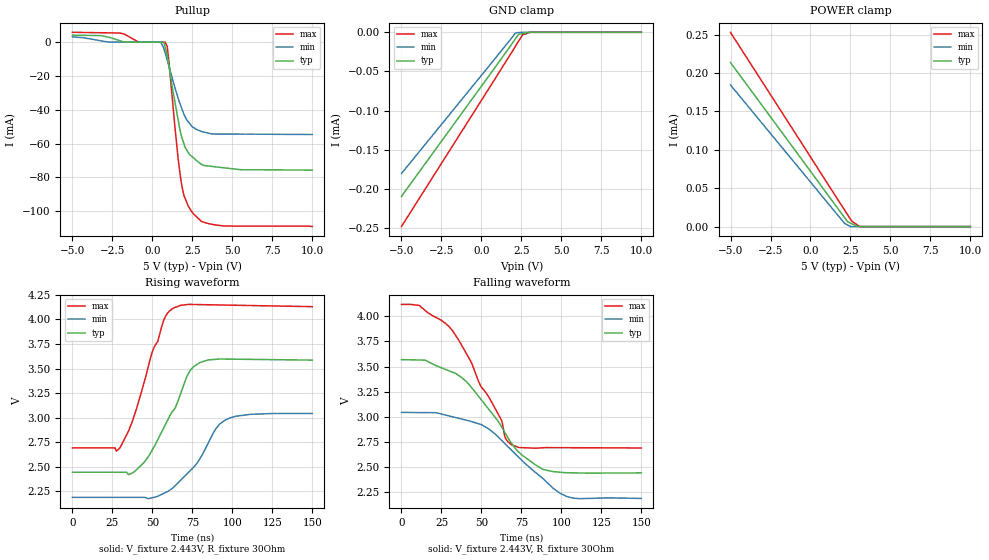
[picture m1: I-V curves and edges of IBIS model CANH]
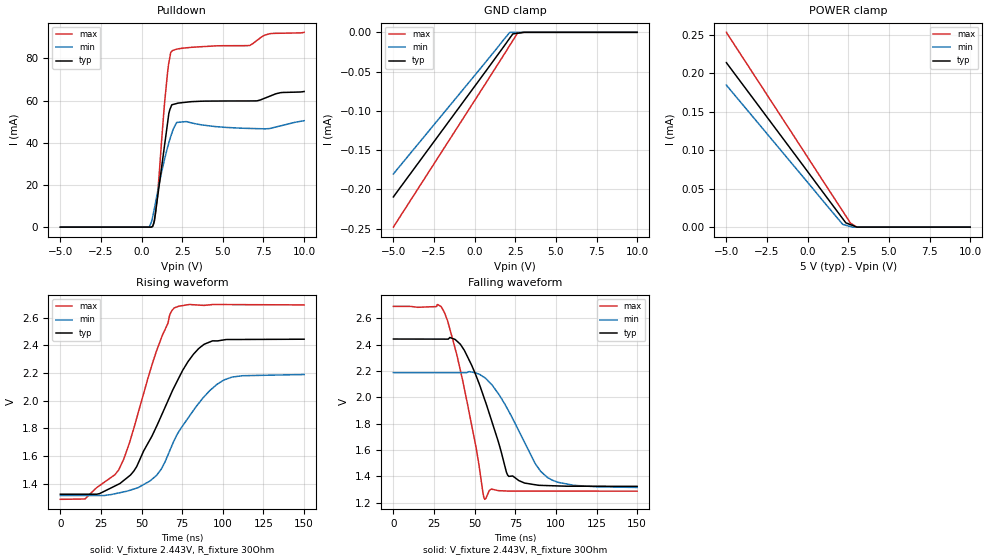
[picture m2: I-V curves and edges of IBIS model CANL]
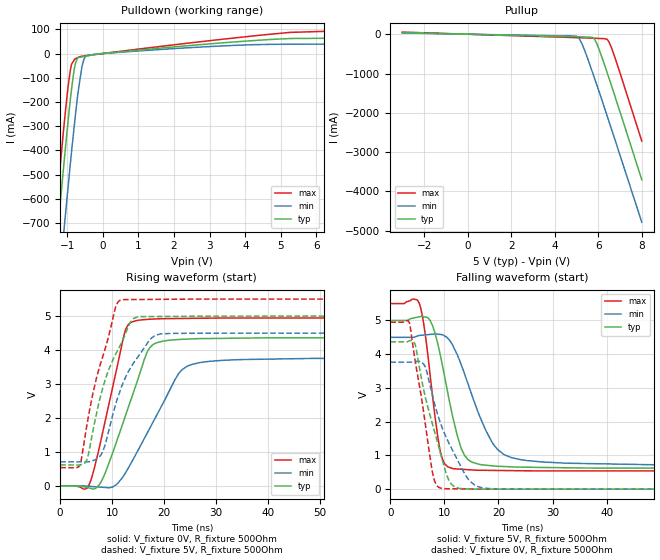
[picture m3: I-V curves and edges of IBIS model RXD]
|Texas Instruments Incorporated
|Automotive Fault Protected CAN Transceiver With Flexible Data-Rate
|Marketing part#   Digital Voltage Range   Package-type   #pins
|TCAN1044D   4.5-5.5V   SOIC   8
[IBIS Ver]   3.2
[File name]   tcan1044-q1.ibs
[File Rev]   1.0
[Date]   11/06/2019
[Source]
| Texas Instruments Incorporated.
| 12500 TI Blvd
| Dallas, TX -75243
[Notes]   Revision History:
| Rev 1.0: 11/06/2019
| - Initial version of the model
| - Model generated from simulations in SPECTRE
| - Model matched to SPICE simulation
| - C_comp although listed in numerical order of value are
|   obtained from varying PVT conditions. For PVT conditions for
|   each specific value refer the buffer description under
|   respective [Model]. IBIS model user is responsible for using
|   appropriate C_comp to simulate for Signal Integrity.
| - Warnings regarding combined Non-monotonicity of various models have been
| reviewed and considered minor and can be ignored.
|* EXCEPTION:   *
|* - For models RXD pullup and pulldown IV curves do not pass   *
|*   through zero because of resistors connected to pad.   *
|* - For CANH model pullup table does not pass through zero   *
|*   due to resistor network connected to PAD. Power clamp table has   *
|*   leakage due to resistor network connected to PAD   *
|* - For CANL model pulldown table does not pass through zero   *
|*   due to resistor network connected to PAD. Power clamp table has   *
|*   leakage due to resistor network connected to PAD   *
[Disclaimer]
| This model is designed as an aid for customers of Texas Instruments.
| TI and its licensors and suppliers make no warranties, either expressed
| or implied, with respect to this  model, including the warranties of
| merchantability or fitness for a particular purpose. The model is
| provided solely on an "as is" basis. The entire risk as to its quality
| and performance is with the customer.
[Copyright]
(C) Copyright 2019 Texas Instruments Incorporated.All rights reserved.
|   TCAN1044D
[Component]   TCAN1044D
[Manufacturer]   TI
[Package]   |8 SOIC - D Package
|   typ   min   max
R_pkg   0.068   0.038   0.098
L_pkg   2.235nH   1.713nH   2.756nH
C_pkg   0.393pF   0.337pF   0.449pF
[Pin]  signal_name   model_name   R_pin   L_pin   C_pin
1   TXD   TXD   0.093   2.653n   0.337p
2   GND   GND   0.038   1.716n   0.449p
3   VCC   POWER   0.038   1.713n   0.449p
4   RXD   RXD   0.093   2.657n   0.337p
5   VIO   POWER   0.098   2.756n   0.341p
6   CANL   CANL   0.092   2.624n   0.363p
7   CANH   CANH   0.075   2.301n   0.349p
8   STB   STB   0.094   2.677n   0.338p
[Diff_pin]   inv_pin   vdiff   tdelay_typ   tdelay_min   tdelay_max
7   6   NA   NA   NA   NA
| Models and submodels in the file (5): CANH (I/O_open_source), CANL (I/O_open_drain), RXD (Output), STB (Input), TXD (Input)
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|   CANH Model
[Model]   CANH
Model_type   I/O_open_source
Polarity   Inverting
Enable   Active-Low
Vinl = 0.5
Vinh = 0.9
Vmeas = 3
Vref = 2.443
Cref = 2pF
Rref = 30
|   typ   min   max
C_comp   12.2e-12   11.49e-12   12.57e-12
[Voltage Range]   5   4.5   5.5
[Temperature Range]   25   150   -55
[Pullup Reference]   5   4.5   5.5
[Pulldown Reference]   0   0   0
[Power Clamp Reference]   5   4.5   5.5
[GND Clamp Reference]   0   0   0
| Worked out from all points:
|   slope of the pullup table from 0 to 0.75 V, typ, clamps not added: 727 ohm
|   falling waveform, V_fixture 2.443V, R_fixture 30Ohm: 20-80 % time 31.2ns typ, 35.1ns min, 29.3ns max; typ from 3.57 V to 2.44 V
|   rising waveform, V_fixture 2.443V, R_fixture 30Ohm: 20-80 % time 20.2ns typ, 21.6ns min, 16.6ns max; typ from 2.44 V to 3.59 V
[GND Clamp]
|   Voltage   I(typ)   I(min)   I(max)
-5V       -209.7uA   -180.5uA   -248.2uA
2.128V    -8.187uA   -910.9nA   -17.7uA
2.322V    -2.722uA   -432nA     -11.25uA
2.569V    -1.686uA   0A         -3.295uA
3.064V    0A         0A         0A
10V       0A         0A         0A
[Pullup]
|   Voltage   I(typ)   I(min)   I(max)
-5V       4.168mA    3.187mA    5.861mA
-2.061V   962.1uA    55.5uA     5.435mA
-861.1mV  8.134uA    7.958uA    128.5uA
482.5mV   3.073uA    -99.63uA   3.64uA
797.2mV   -2.85mA    -6.239mA   -7.214uA
930.8mV   -8.028mA   -10.68mA   -2.658mA
1.594V    -45.06mA   -32.61mA   -67.39mA
1.848V    -56.59mA   -39.51mA   -85.28mA
2.229V    -65.02mA   -46.88mA   -96.72mA
3.064V    -72.18mA   -52.81mA   -106mA
4.442V    -74.24mA   -54.38mA   -108.7mA
10V       -75.66mA   -54.59mA   -109mA
[POWER Clamp]
|   Voltage   I(typ)   I(min)   I(max)
-5V       213.6uA    184.5uA    252.9uA
2.128V    11.78uA    4.269uA    21.63uA
2.322V    6.298uA    2.025uA    15.35uA
2.569V    3.9uA      0A         7.37uA
3.064V    0A         0A         0A
10V       0A         0A         0A
[Ramp]
R_load = 30
|   typ   min   max
dV/dt_r   0.685442/2.00542e-08   0.512592/2.14191e-08   0.863536/1.66139e-08
dV/dt_f   0.674704/3.11586e-08   0.512317/3.5057e-08   0.855212/2.92131e-08
[Falling Waveform]
V_fixture = 2.443V
V_fixture_min = 2.188V
V_fixture_max = 2.691V
R_fixture = 30Ohm
C_fixture = 0F
|   Time   V(typ)   V(min)   V(max)
0s        3.569V     3.045V     4.117V
11.28ns   3.565V     3.043V     4.106V
31.67ns   3.445V     3.002V     3.861V
50.06ns   3.167V     2.923V     3.294V
62.3ns    2.909V     2.772V     2.975V
64.87ns   2.84V      2.731V     2.793V
68.51ns   2.745V     2.674V     2.726V
88.48ns   2.479V     2.388V     2.694V
103.4ns   2.446V     2.21V      2.694V
150ns     2.444V     2.191V     2.691V
[Rising Waveform]
V_fixture = 2.443V
V_fixture_min = 2.188V
V_fixture_max = 2.691V
R_fixture = 30Ohm
C_fixture = 0F
|   Time   V(typ)   V(min)   V(max)
0s        2.443V     2.188V     2.691V
29.42ns   2.443V     2.188V     2.686V
37.65ns   2.437V     2.188V     2.97V
45.02ns   2.548V     2.188V     3.371V
57.13ns   2.897V     2.228V     3.994V
62.96ns   3.071V     2.285V     4.115V
75.77ns   3.519V     2.493V     4.153V
89.67ns   3.594V     2.888V     4.148V
95.81ns   3.596V     2.978V     4.147V
150ns     3.586V     3.042V     4.13V
|   CANL Model
[Model]   CANL
Model_type   I/O_open_drain
Polarity   Non-Inverting
Enable   Active-Low
Vinl = 0.5
Vinh = 0.9
Vmeas = 2
Vref = 2.443
Cref = 2pF
Rref = 30
|   typ   min   max
C_comp   11.96e-12   11.44e-12   12.21e-12
[Voltage Range]   5   4.5   5.5
[Temperature Range]   25   150   -55
[Pullup Reference]   5   4.5   5.5
[Pulldown Reference]   0   0   0
[Power Clamp Reference]   5   4.5   5.5
[GND Clamp Reference]   0   0   0
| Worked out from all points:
|   slope of the pulldown table from 0 to 0.75 V, typ, clamps not added: 373 ohm
|   falling waveform, V_fixture 2.443V, R_fixture 30Ohm: 20-80 % time 18.1ns typ, 22.3ns min, 14.4ns max; typ from 2.44 V to 1.32 V
|   rising waveform, V_fixture 2.443V, R_fixture 30Ohm: 20-80 % time 27.4ns typ, 26.3ns min, 22.2ns max; typ from 1.32 V to 2.44 V
[Pulldown]
|   Voltage   I(typ)   I(min)   I(max)
-5V       30fA       -53.22pA   460fA
252.8mV   4.719uA    -3.121uA   -1.871uA
647.3mV   194.8uA    3.573mA    145.6uA
782.7mV   2.825mA    8.677mA    2.945mA
979mV     13.95mA    16.53mA    15.09mA
1.407V    38.49mA    32.05mA    58.45mA
1.6V      49.55mA    37.9mA     73.56mA
1.894V    58.11mA    45.29mA    83.7mA
2.755V    59.27mA    50.08mA    85.07mA
6.669V    59.86mA    46.81mA    86.22mA
7.601V    61.23mA    46.63mA    91.14mA
10V       64.34mA    50.49mA    92.41mA
[GND Clamp]
|   Voltage   I(typ)   I(min)   I(max)
-5V       -209.7uA   -180.5uA   -248.2uA
2.155V    -7.531uA   -153.4nA   -16.77uA
2.349V    -2.037uA   -103.9nA   -10.51uA
2.638V    -1.181uA   -29.97nA   -1.117uA
3.037V    0A         0A         0A
10V       0A         0A         0A
[POWER Clamp]
|   Voltage   I(typ)   I(min)   I(max)
-5V       213.6uA    184.5uA    252.9uA
2.155V    11.02uA    3.595uA    20.77uA
2.349V    5.558uA    2.436uA    14.52uA
2.638V    3.222uA    702.3nA    5.157uA
3.031V    53.18nA    0A         0A
10V       0A         0A         0A
[Ramp]
R_load = 30
|   typ   min   max
dV/dt_r   0.671493/2.72876e-08   0.524178/2.61335e-08   0.842197/2.20483e-08
dV/dt_f   0.671494/1.80697e-08   0.523421/2.22127e-08   0.842202/1.44627e-08
[Falling Waveform]
V_fixture = 2.443V
V_fixture_min = 2.188V
V_fixture_max = 2.691V
R_fixture = 30Ohm
C_fixture = 0F
|   Time   V(typ)   V(min)   V(max)
0s        2.443V     2.188V     2.691V
27.22ns   2.443V     2.188V     2.706V
31.4ns    2.443V     2.188V     2.646V
41.22ns   2.404V     2.188V     2.205V
56.2ns    1.983V     2.15V      1.226V
60.2ns    1.832V     2.101V     1.303V
71.01ns   1.4V       1.894V     1.288V
87.3ns    1.336V     1.497V     1.288V
94.67ns   1.33V      1.393V     1.288V
150ns     1.324V     1.316V     1.288V
[Rising Waveform]
V_fixture = 2.443V
V_fixture_min = 2.188V
V_fixture_max = 2.691V
R_fixture = 30Ohm
C_fixture = 0F
|   Time   V(typ)   V(min)   V(max)
0s        1.324V     1.315V     1.288V
15.16ns   1.324V     1.315V     1.29V
35.89ns   1.397V     1.334V     1.5V
45.28ns   1.493V     1.362V     1.803V
59.14ns   1.813V     1.46V      2.358V
67.49ns   2.033V     1.643V     2.626V
70ns      2.097V     1.711V     2.668V
85.22ns   2.377V     1.982V     2.69V
100.8ns   2.439V     2.15V      2.694V
150ns     2.444V     2.189V     2.691V
|   RXD Model
[Model]   RXD
Model_type   Output
Polarity   Non-Inverting
Vmeas = 2.5
Vref = 0
Cref = 2pF
Rref = 500
|   typ   min   max
C_comp   6.425e-12   6.1e-12   6.5e-12
[Voltage Range]   5   4.5   5.5
[Temperature Range]   25   150   -55
[Pullup Reference]   5   4.5   5.5
[Pulldown Reference]   0   -0   0
[Power Clamp Reference]   5   4.5   5.5
[GND Clamp Reference]   0   0   0
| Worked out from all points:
|   slope of the pulldown table from 0 to 0.75 V, typ, clamps not added: 70.6 ohm
|   slope of the pullup table from 0 to 0.75 V, typ, clamps not added: 72.7 ohm
|   falling waveform, V_fixture 5V, R_fixture 500Ohm: 20-80 % time 3.52ns typ, 5.58ns min, 2.28ns max; typ from 5 V to 0.617 V
|   rising waveform, V_fixture 0V, R_fixture 500Ohm: 20-80 % time 5.84ns typ, 7.77ns min, 4.28ns max; typ from 0 V to 4.37 V
|   rising waveform, V_fixture 5V, R_fixture 500Ohm: 20-80 % time 5.36ns typ, 5.61ns min, 4.62ns max; typ from 0.617 V to 5 V
|   falling waveform, V_fixture 0V, R_fixture 500Ohm: 20-80 % time 4.11ns typ, 5.33ns min, 2.86ns max; typ from 4.37 V to 0 V
[Pulldown]
|   Voltage   I(typ)   I(min)   I(max)
-3V       -3.693A    -3.921A    -3.585A
-1.522V   -1.154A    -1.425A    -1.005A
-1.302V   -788.4mA   -1.065A    -633.8mA
-1.082V   -436.3mA   -713.9mA   -282mA
-972mV    -271.3mA   -544.6mA   -129.8mA
-889.5mV  -158.8mA   -420.6mA   -51.01mA
-793.3mV  -56.55mA   -285.1mA   -23.42mA
-710.8mV  -17.01mA   -176.8mA   -17.28mA
-587mV    -13.6mA    -53.55mA   -11.33mA
-449.1mV  -9.808mA   -7.528mA   -8.666mA
5.265V    61.92mA    38.42mA    87.41mA
8V        64.79mA    47.59mA    99.6mA
[Pullup]
|   Voltage   I(typ)   I(min)   I(max)
-3V       41.95mA    32.12mA    53.99mA
5.051V    -66.26mA   -65.41mA   -88.43mA
5.134V    -67.25mA   -115.4mA   -89.83mA
5.368V    -70.05mA   -400.3mA   -93.78mA
5.746V    -82.06mA   -988.6mA   -101.5mA
5.822V    -118.5mA   -1.11A     -103.2mA
6.022V    -362.1mA   -1.434A    -107.6mA
6.407V    -973.2mA   -2.075A    -131.6mA
6.489V    -1.11A     -2.214A    -190.6mA
6.603V    -1.3A      -2.405A    -337.5mA
6.962V    -1.911A    -3.012A    -916.7mA
8V        -3.701A    -4.781A    -2.718A
[Ramp]
R_load = 500
|   typ   min   max
dV/dt_r   2.61984/5.84173e-09   2.25875/7.76556e-09   2.96883/4.28243e-09
dV/dt_f   2.63008/3.50076e-09   2.27668/5.55338e-09   2.97767/2.27363e-09
[Falling Waveform]
V_fixture = 5V
V_fixture_min = 4.5V
V_fixture_max = 5.5V
R_fixture = 500Ohm
C_fixture = 0F
|   Time   V(typ)   V(min)   V(max)
0s        5V         4.5V       5.5V
5.348ns   5.108V     4.556V     5.512V
6.135ns   5.111V     4.568V     4.937V
7.406ns   4.984V     4.588V     3.317V
9.185ns   4.017V     4.587V     1.16V
11.49ns   2.175V     4.277V     613.1mV
14.48ns   861.3mV    3.065V     576.3mV
19.21ns   686.3mV    1.296V     555.3mV
24.36ns   652.4mV    868mV      546.1mV
150ns     616.5mV    705.5mV    537.2mV
[Rising Waveform]
V_fixture = 0V
V_fixture_min = 0V
V_fixture_max = 0V
R_fixture = 500Ohm
C_fixture = 0F
|   Time   V(typ)   V(min)   V(max)
0s        -18.78nV   -44.31nV   16.35nV
5.65ns    -66.98mV   -14.2mV    64.05mV
8.191ns   211.8mV    -42.83mV   1.58V
12.39ns   1.988V     338.3mV    4.503V
14.48ns   2.919V     903.1mV    4.859V
16.66ns   3.912V     1.53V      4.9V
17.75ns   4.146V     1.844V     4.91V
22.9ns    4.31V      3.326V     4.928V
27.33ns   4.335V     3.64V      4.936V
150ns     4.366V     3.765V     4.948V
[Rising Waveform]
V_fixture = 5V
V_fixture_min = 4.5V
V_fixture_max = 5.5V
R_fixture = 500Ohm
C_fixture = 0F
|   Time   V(typ)   V(min)   V(max)
0s        616.5mV    705.5mV    537.2mV
3.852ns   614.1mV    706.5mV    622.1mV
5.252ns   816.1mV    706.8mV    1.877V
7.911ns   2.721V     926mV      3.667V
10.72ns   3.886V     2.419V     5.286V
11.89ns   4.235V     2.95V      5.481V
14.13ns   4.929V     3.621V     5.486V
17.37ns   4.984V     4.326V     5.49V
19.77ns   4.987V     4.48V      5.492V
150ns     5V         4.5V       5.5V
[Falling Waveform]
|GND
V_fixture = 0V
V_fixture_min = 0V
V_fixture_max = 0V
R_fixture = 500Ohm
C_fixture = 0F
|   Time   V(typ)   V(min)   V(max)
0s        4.366V     3.765V     4.948V
3.549ns   4.402V     3.764V     4.921V
4.645ns   4.257V     3.778V     3.744V
6.24ns    2.893V     3.688V     2.186V
7.819ns   1.915V     2.763V     475mV
9.547ns   910mV      1.838V     17.76mV
11.91ns   67.79mV    1.023V     10.82mV
14.64ns   4.995mV    248.9mV    5.801mV
17.56ns   3.25mV     26.21mV    1.003mV
150ns     -139.7nV   277.6nV    -3.082nV
